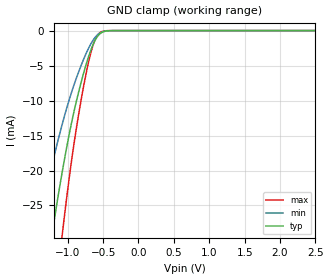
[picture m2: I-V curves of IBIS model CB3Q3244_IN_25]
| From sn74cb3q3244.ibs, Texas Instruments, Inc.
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[Model]   CB3Q3244_IN_25
Model_type  Input
Vinl=0.7
Vinh=1.7
| variable   typ   min   max
C_comp   1.72pF   1.36pF   1.89pF
[Temperature Range]   40   100   -40
| Ambient temperature   25   85   -40
[Voltage range]   2.5   2.3   2.7
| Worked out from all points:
|   GND clamp passes 1 mA (typ) near -0.59 V on its own axis
[GND Clamp]
| CB3Q3244_IN_25
|   Voltage   I(typ)   I(min)   I(max)
-5.5V     -449.4mA   -341.7mA   -564.9mA
-1.43V    -44.05mA   -29.14mA   -63.84mA
-1.385V   -40.69mA   -26.88mA   -59.08mA
-1.21V    -28.44mA   -18.75mA   -41.42mA
-1.075V   -20.08mA   -13.3mA    -29.01mA
-930mV    -12.45mA   -8.348mA   -17.51mA
-780mV    -6.266mA   -4.228mA   -8.232mA
-705mV    -3.722mA   -2.522mA   -4.498mA
-650mV    -2.201mA   -1.506mA   -2.36mA
-550mV    -508.6uA   -385.4uA   -338.8uA
-350mV    -3.427uA   -5.101uA   -376.5nA
2.5V      153pA      445.6pA    85.38pA
